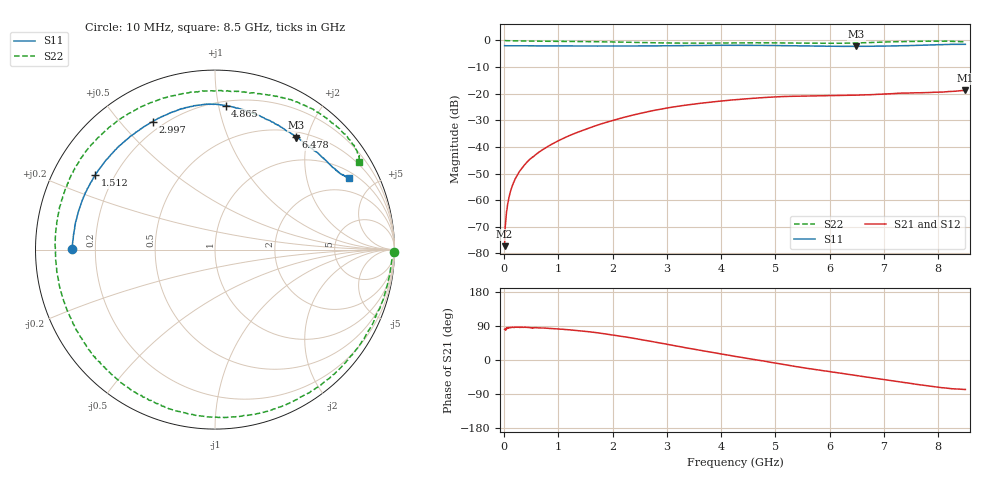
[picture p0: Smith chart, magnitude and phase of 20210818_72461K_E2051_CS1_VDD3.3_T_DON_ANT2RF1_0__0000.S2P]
!Agilent Technologies,E5071C,MY46417908,A.11.23
!Date: Wed Aug 18 14:22:46 2021
!Data & Calibration Information:
!Freq	S11:SOLT2(ON)	S21:SOLT2(ON)	S12:SOLT2(ON)	S22:SOLT2(ON)
!PortZ  Port1:50+j0  Port2:50+j0
!Above PortZ is port z conversion or system Z0 setting when saving the data.
!When reading, reference impedance value at option line is always used.
# Hz S dB R 50
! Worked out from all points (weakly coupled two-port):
!   1601 points, 10 MHz to 8.5 GHz, reference 50 ohm
!   highest |S21| = -18.78 dB at 8.495 GHz (marker M1); lowest = -77.3 dB at 10 MHz (marker M2)
!   lowest |S11| = -2.3 dB at 6.489 GHz (marker M3), VSWR 7.75, Z = 29.4 + j90.7 ohm
!   |S11| at or under -10 dB: nowhere
!   |S22| runs from -1.1 to 0.0 dB; largest |S21 - S12| = 0.00049
!   S11 on the Smith chart (normalised r, x): 10 MHz: 0.11, +0.00; 1.512 GHz: 0.13, +0.28; 2.997 GHz: 0.16, +0.61; 4.865 GHz: 0.23, +1.05; 6.478 GHz: 0.58, +1.80; 8.5 GHz: 1.28, +3.56
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1e7  -1.96 179.7  -77.27 81.0  -77.13 79.7  -0.01 -0.6
6.836875e7  -2.00 178.5  -61.31 85.6  -61.34 84.5  -0.11 -3.3
1.108188e8  -2.00 177.7  -57.21 85.7  -57.20 85.8  -0.13 -5.2
1.957188e8  -2.02 175.8  -52.47 86.0  -52.52 86.4  -0.15 -8.8
3.177625e8  -2.03 173.2  -48.22 86.3  -48.24 86.6  -0.19 -14.2
4.822562e8  -2.03 169.8  -44.58 85.2  -44.59 85.4  -0.26 -21.2
7.475688e8  -2.04 164.1  -40.55 84.2  -40.55 84.3  -0.30 -32.4
1.426769e9  -2.09 149.8  -33.95 76.5  -33.96 76.4  -0.44 -62.1
1.511669e9  -2.09 147.9  -33.33 75.3  -33.32 75.3  -0.45 -65.8
2.180256e9  -2.10 133.4  -29.04 62.2  -29.05 62.3  -0.64 -97.2
2.843538e9  -2.03 119.2  -25.97 45.7  -25.98 45.7  -0.89 -131.4
2.997419e9  -2.01 116.0  -25.42 41.7  -25.41 41.7  -0.95 -139.5
3.61825e9  -1.88 104.6  -23.60 25.4  -23.59 25.6  -1.02 -172.0
4.255e9  -1.83 94.8  -22.27 9.7  -22.29 9.8  -0.92 157.6
4.865219e9  -1.89 85.8  -21.33 -4.8  -21.35 -4.8  -0.91 131.7
5.671769e9  -2.09 71.8  -20.85 -23.7  -20.85 -23.7  -1.04 101.7
6.478319e9  -2.25 54.3  -20.58 -40.8  -20.59 -40.8  -0.98 77.9
6.488931e9  -2.25 54.0  -20.59 -41.0  -20.60 -41.0  -0.98 77.6
7.088538e9  -2.07 41.8  -20.05 -53.4  -20.09 -53.6  -0.57 62.4
7.937538e9  -1.65 30.2  -19.46 -70.7  -19.44 -70.7  -0.28 40.8
8.494694e9  -1.46 28.1  -18.78 -77.7  -18.79 -77.9  -0.53 31.5
8.5e9  -1.47 28.2  -18.78 -77.7  -18.79 -77.8  -0.55 31.3
